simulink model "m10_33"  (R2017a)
settings: Solver=ode45  StartTime=0.0  StopTime=20.0  RelTol=1e-3  EnableMultiTasking=on
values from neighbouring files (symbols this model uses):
  beta = 5    [ini_mst.m]    (also in vdpini.m = sqrt(3))
  omega = 4    [ini_mst.m]    (also in vdpini.m = 1)
  x01 = 50    [ini_mst.m]
  x02 = 0    [ini_mst.m]

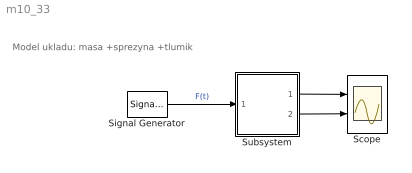
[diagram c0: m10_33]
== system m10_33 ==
  note: Model ukladu: masa +sprezyna +tlumik
  Scope : Scope  NumInputPorts=2
  Signal Generator : SignalGenerator  Amplitude=0
  Subsystem : Subsystem
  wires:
  Signal Generator/1 -> Subsystem/1(In1)  "F(t)"
  Subsystem/1(Out1) -> Scope/1
  Subsystem/2(Out2) -> Scope/2

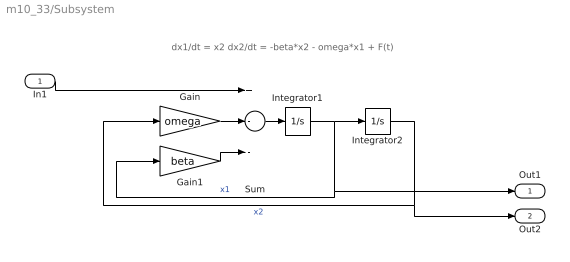
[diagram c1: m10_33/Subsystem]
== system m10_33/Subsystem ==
  note: dx1/dt = x2 dx2/dt = -beta*x2 - omega*x1 + F(t)
  In1 : Inport
  Gain : Gain  Gain=omega
  Gain1 : Gain  Gain=beta
  Integrator1 : Integrator  InitialCondition=x01
  Integrator2 : Integrator  InitialCondition=x02
  Sum : Sum  Inputs=+--
  Out1 : Outport
  Out2 : Outport  Port=2
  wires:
  Gain/1 -> Sum/2
  Integrator2/1 -> Out2/1, Gain/1  "x2"
  Sum/1 -> Integrator1/1
  Gain1/1 -> Sum/3
  Integrator1/1 -> Out1/1, Gain1/1, Integrator2/1  "x1"
  In1/1 -> Sum/1
